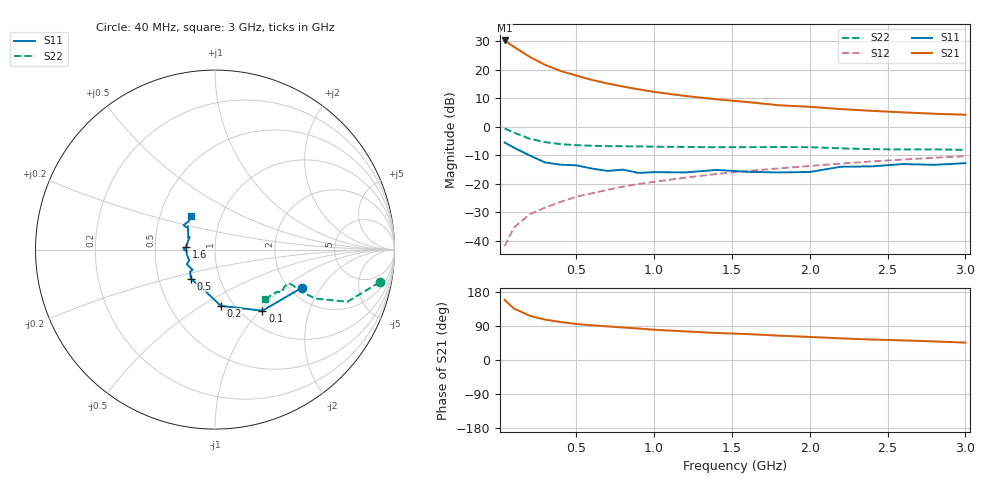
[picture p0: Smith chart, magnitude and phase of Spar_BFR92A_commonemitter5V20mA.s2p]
! Filename:  BFR92AE.S2P  Version:  2.0
! NXP part #: BFR92A  Date: May 1990
! Bias condition: Vce=5V, Ic=20mA
#  MHz  S  MA  R  50
! Freq  S11  S21  S12  S22  !GUM [dB]
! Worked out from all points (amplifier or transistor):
!   21 points, 40 MHz to 3 GHz, reference 50 ohm
!   highest |S21| = 30.4 dB at 40 MHz (marker M1)
!   |S21| within 3 dB of that: start of sweep to 122.1 MHz
!   unconditionally stable (mu >= 1): 654 MHz to 777.7 MHz; 816.5 MHz to 2.507 GHz
!   at 300 MHz: K = 0.87, MSG = 25.1 dB, |S12| = -28.4 dB
!   at 1 GHz: K = 1.03, MAG = 14.8 dB, |S12| = -19.3 dB
!   at 3 GHz: K = 0.98, MSG = 7.3 dB, |S12| = -10.3 dB
!   S11 on the Smith chart (normalised r, x): 40 MHz: 2.33, -1.37; 100 MHz: 1.24, -1.04; 200 MHz: 0.87, -0.61; 500 MHz: 0.73, -0.25; 1.6 GHz: 0.72, +0.02; 3 GHz: 0.71, +0.28
40  0.53 -23.5  32.95 158.4  0.008 79.3  0.935 -11.2
100  0.431 -52.2  25.49 135.8  0.017 72.0  0.793 -21.5
200  0.315 -84.1  17.06 117.0  0.029 69.1  0.619 -26.1
300  0.237 -103.4  12.28 106.5  0.038 71.7  0.538 -25.8
400  0.216 -116.9  9.567 100.3  0.048 73.2  0.497 -25.2
500  0.211 -129.8  7.971 95.0  0.059 74.5  0.476 -24.6
600  0.185 -138.4  6.68 91.7  0.068 74.5  0.465 -24.6
700  0.168 -138.1  5.788 88.7  0.078 76.0  0.458 -24.7
800  0.177 -152.4  5.103 85.8  0.089 75.3  0.456 -24.9
900  0.155 -157.8  4.57 83.1  0.099 76.5  0.453 -25.2
1000  0.16 -170.5  4.115 79.9  0.108 76.8  0.448 -25.4
1200  0.158 -176.4  3.488 75.5  0.128 76.0  0.443 -26.7
1400  0.175 179.7  3.048 71.3  0.148 75.0  0.438 -28.6
1600  0.162 174.3  2.725 68.4  0.168 75.1  0.44 -30.1
1800  0.158 153.5  2.397 64.3  0.186 74.3  0.441 -31.8
2000  0.161 157.3  2.248 60.9  0.205 73.2  0.439 -32.9
2200  0.199 139.4  2.054 57.1  0.226 72.8  0.419 -34.0
2400  0.202 142.0  1.907 54.0  0.247 71.2  0.405 -37.7
2600  0.222 142.3  1.798 51.8  0.266 70.2  0.4 -41.4
2800  0.215 132.7  1.699 49.0  0.286 69.6  0.402 -43.9
3000  0.23 126.3  1.632 45.9  0.305 68.1  0.394 -44.8
